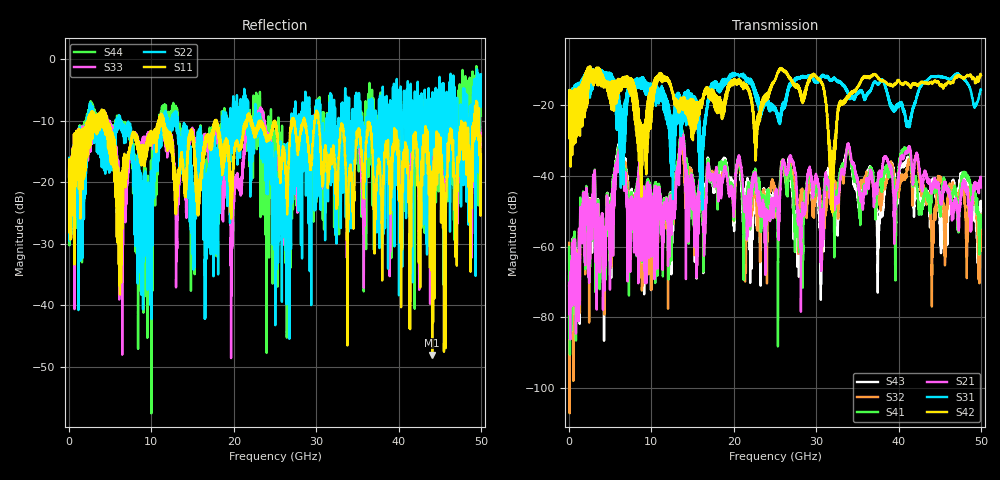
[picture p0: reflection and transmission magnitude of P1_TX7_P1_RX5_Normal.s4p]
!Keysight Technologies,N5225B,MY57041031,A.13.20.10
!Date: Friday, May 31, 2019 11:21:10
!Correction: S11(Full 4 Port(1,2,3,4))
!S12(Full 4 Port(1,2,3,4))
!S13(Full 4 Port(1,2,3,4))
!S14(Full 4 Port(1,2,3,4))
!S21(Full 4 Port(1,2,3,4))
!S22(Full 4 Port(1,2,3,4))
!S23(Full 4 Port(1,2,3,4))
!S24(Full 4 Port(1,2,3,4))
!S31(Full 4 Port(1,2,3,4))
!S32(Full 4 Port(1,2,3,4))
!S33(Full 4 Port(1,2,3,4))
!S34(Full 4 Port(1,2,3,4))
!S41(Full 4 Port(1,2,3,4))
!S42(Full 4 Port(1,2,3,4))
!S43(Full 4 Port(1,2,3,4))
!S44(Full 4 Port(1,2,3,4))
!S4P File: Measurements: <S11,S12,S13,S14>,
!<S21,S22,S23,S24>,
!<S31,S32,S33,S34>,
!<S41,S42,S43,S44>:
# Hz S  dB  R 50.0
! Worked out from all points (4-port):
!   5000 points, 10 MHz to 50 GHz, reference 50 ohm
!   strongest paths, dB at 10 MHz, 12.51 GHz, 25.01 GHz, 37.51 GHz, 50 GHz:
!     S42: -19.5, -15.6, -12.9, -12.4, -11.5
!     S31: -19.4, -39.6, -20.8, -14.0, -15.5
!     S21: -71.0, -48.5, -44.9, -41.1, -43.3
!     S41: -60.1, -50.6, -47.2, -41.2, -52.9
!     S32: -59.0, -50.3, -45.4, -46.1, -56.4
!     S43: -68.4, -55.5, -43.6, -64.1, -49.5
!   lowest |S11| = -48.1 dB at 44.09 GHz (marker M1), VSWR 1.01, Z = 49.7 + j0.271 ohm
!   |S11| at or under -10 dB: 4.613 GHz to 10.86 GHz (6.246 GHz wide, 80.7 % of centre); 11.46 GHz to 17.74 GHz (6.279 GHz wide, 43 % of centre); 30.28 GHz to 47.62 GHz (17.34 GHz wide, 44.5 % of centre)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
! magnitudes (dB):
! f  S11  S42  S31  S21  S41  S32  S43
! 10 MHz  -19.1  -19.5  -19.4  -71.0  -60.1  -59.0  -68.4
! 6.23 GHz  -30.7  -13.6  -23.6  -31.8  -31.0  -31.1  -30.3
! 9.04 GHz  -14.5  -28.9  -13.3  -46.4  -54.7  -51.8  -61.6
! 29.79 GHz  -10.0  -11.2  -13.4  -42.0  -45.9  -47.6  -45.8
! 31.91 GHz  -16.7  -46.5  -12.8  -38.9  -37.9  -46.0  -38.0
! 44.09 GHz  -48.1  -13.9  -11.8  -42.8  -43.1  -59.4  -41.5
! 50 GHz  -15.5  -11.5  -15.5  -43.3  -52.9  -56.4  -49.5
